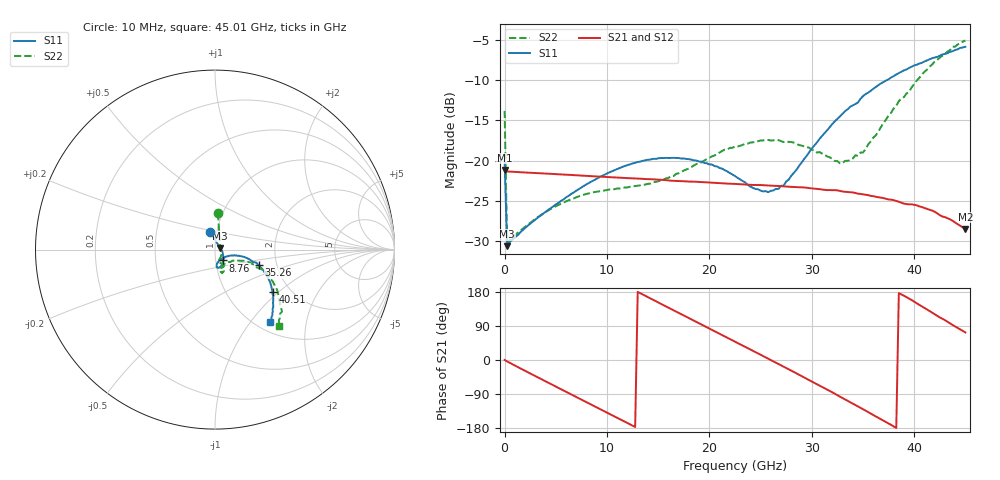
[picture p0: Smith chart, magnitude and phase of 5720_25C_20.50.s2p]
! Device:  ADRF5720
! Description: 0.5dB LSB GaAs MMIC 6-bit Digital Attenuator
! Frequency:  0.000009 -  40 GHz
! Ports:
!	RF1	= Port 1
!	RF2	= Port 2
! Vdd:  3.3 Volt
! Vss:  -3.3 Volt
! Control:  0/3.3 Volt
! State:  20.50 dB attenuation
! Data:  The device was measured using G-S-G Probes on a matrix board.
!  Data was collected using an calibrated 4 port network analyzer.
!  The reference plane for this measurement is at the launchers.
! Note:  Analog Devices supplies this data as a sample of measured data
!  for this product.  Your particular data for this product may vary.
!  Data was taken at 25 degrees C.
!  Analog Devices reserves the right to change this data at anytime.
# GHZ S DB R 45.0
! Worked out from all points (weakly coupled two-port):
!   181 points, 10 MHz to 45.01 GHz, reference 45 ohm
!   highest |S21| = -21.15 dB at 10 MHz (marker M1); lowest = -28.5 dB at 45.01 GHz (marker M2)
!   lowest |S11| = -30.6 dB at 260 MHz (marker M3), VSWR 1.06, Z = 47.6 + j0.86 ohm
!   |S11| at or under -10 dB: start of sweep to 37.37 GHz
!   |S22| runs from -30.5 to -5.1 dB; largest |S21 - S12| = 0.00017
!   S11 on the Smith chart (normalised r, x): 10 MHz: 0.93, +0.18; 8.76 GHz: 1.09, -0.13; 35.26 GHz: 1.61, -0.30; 40.51 GHz: 1.62, -0.92; 45.01 GHz: 1.15, -1.26
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0.01  -20.06 104.8  -21.15 0.1  -21.15 0.1  -13.83 85.3
0.26  -30.61 17.8  -21.35 -3.9  -21.35 -3.9  -30.47 15.1
1.26  -29.28 0.4  -21.42 -18.1  -21.42 -18.1  -28.98 -8.1
3.51  -26.82 -21.0  -21.57 -49.4  -21.57 -49.4  -26.79 -38.0
7.76  -23.13 -48.1  -21.87 -108.0  -21.87 -108.0  -24.22 -68.3
8.760001  -22.42 -52.8  -21.95 -121.7  -21.94 -121.7  -23.91 -71.6
12.01  -20.55 -66.0  -22.17 -166.4  -22.17 -166.4  -23.32 -75.3
15.26  -19.68 -76.1  -22.38 148.5  -22.38 148.5  -22.44 -70.0
19.26  -20.13 -84.1  -22.66 93.2  -22.66 93.3  -20.21 -63.5
22.76  -22.14 -81.2  -22.91 44.9  -22.91 44.9  -18.25 -65.8
25.26  -23.83 -60.5  -23.05 10.3  -23.05 10.3  -17.50 -70.6
26.76  -23.51 -41.6  -23.15 -10.6  -23.15 -10.6  -17.47 -72.4
27.76  -22.35 -29.5  -23.24 -24.7  -23.24 -24.6  -17.68 -74.1
30.26  -18.13 -15.2  -23.47 -60.4  -23.47 -60.3  -18.74 -73.6
32.76  -14.53 -15.2  -23.76 -96.7  -23.76 -96.7  -20.34 -59.7
33.76  -13.31 -17.1  -23.92 -111.2  -23.92 -111.2  -19.96 -46.9
35.26  -11.75 -19.5  -24.22 -133.7  -24.21 -133.7  -18.58 -31.6
37.76  -9.68 -27.4  -24.84 -171.3  -24.86 -171.2  -14.06 -20.3
40.51  -7.96 -36.6  -25.68 145.4  -25.68 145.5  -9.74 -25.9
42.26  -7.14 -42.7  -26.54 116.2  -26.53 116.2  -7.51 -34.0
43.76  -6.44 -47.9  -27.46 92.4  -27.47 92.5  -5.87 -42.8
45.01  -5.88 -52.9  -28.49 72.7  -28.48 72.8  -5.10 -50.1
